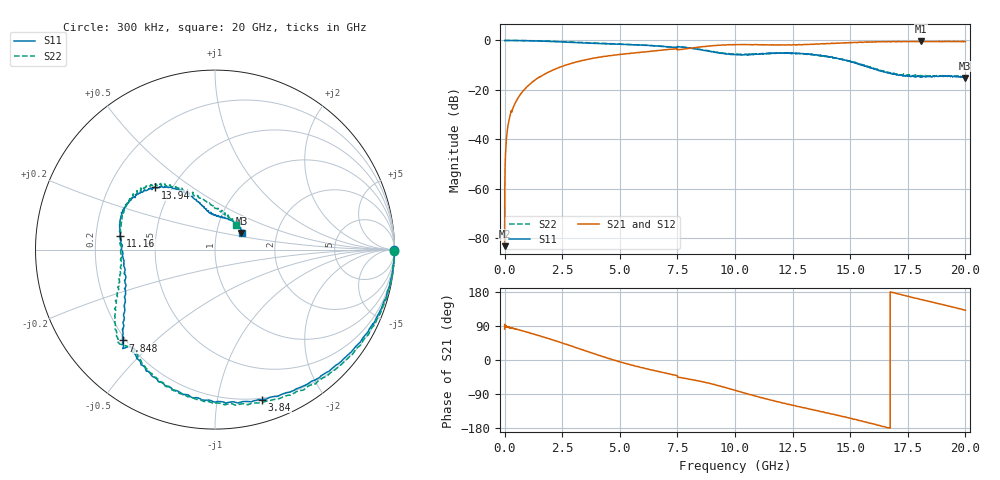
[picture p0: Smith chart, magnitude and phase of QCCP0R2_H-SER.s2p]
!{QCCP0R2}
!Johanson Technology Inc.
!www.johansontechnology.com
!Test Board Conditions:
!Substrate Type  RO4350B
!Substrate Thickness  20 mil
!Substrate Dk  3.66
!TL Type: GCPW
!TL Trace Width  36 mil
!TL Gap  12 mil
!Electrode orientation  Horizontal
!DUT TOPOLOGY	SERIES
!Mounting Pad LxW  26x36 mil
! Created Sat Jan  9 18:23:01 2021
# hz S ma R 50
! 2 Port Network Data from SP1.SP block
! freq  magS11  angS11  magS21  angS21  magS12  angS12  magS22  angS22
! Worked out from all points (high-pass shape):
!   20001 points, 300 kHz to 20 GHz, reference 50 ohm
!   highest |S21| = -0.38 dB at 18.08 GHz (marker M1); lowest = -83.3 dB at 300 kHz (marker M2)
!   |S21| within 3 dB of the highest: 7.476661 GHz to 7.499038 GHz (22.38 MHz wide, 0.299 % of centre); 7.867 GHz to end of sweep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
!   lowest |S11| = -15.2 dB at 20 GHz (marker M3), VSWR 1.42, Z = 65.9 + j12.5 ohm
!   |S11| at or under -10 dB: 15.54 GHz to end of sweep
!   |S22| runs from -14.9 to 0.0 dB; largest |S21 - S12| = 0.011
!   S11 on the Smith chart (normalised r, x): 300 kHz: open; 3.84 GHz: 0.19, -1.35; 7.848 GHz: 0.19, -0.40; 11.16 GHz: 0.30, +0.06; 13.94 GHz: 0.41, +0.36; 20 GHz: 1.32, +0.25
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300000  0.9946 -0.3  6.827e-05 81.7  9.806e-05 134.2  0.9961 -0.3
1.033e8  0.997 -1.7  0.01317 88.1  0.01316 87.8  0.9976 -1.8
1.453e8  0.9998 -2.5  0.01862 87.0  0.01853 87.3  0.9991 -2.5
2.763e8  0.9982 -4.7  0.03533 84.7  0.03533 84.6  0.9983 -4.8
5.343e8  0.9965 -8.5  0.06283 80.9  0.06278 80.9  0.9978 -8.6
9.283e8  0.9903 -15.2  0.1099 74.2  0.1099 74.3  0.9936 -15.3
1.4723e9  0.9754 -24.8  0.1779 64.6  0.1775 64.4  0.9828 -25.1
3.3343e9  0.8968 -61.9  0.3898 27.9  0.389 27.8  0.9132 -62.2
3.8403e9  0.8761 -72.5  0.4359 17.4  0.4347 17.6  0.8899 -72.7
5.2683e9  0.8303 -99.4  0.537 -9.4  0.5353 -9.1  0.8323 -99.5
6.6673e9  0.7732 -119.9  0.6267 -30.1  0.6266 -30.0  0.7679 -119.2
7.8483e9  0.7205 -135.4  0.6767 -48.4  0.6762 -48.6  0.7251 -139.4
8.8633e9  0.6055 -146.2  0.7698 -61.0  0.7687 -61.1  0.6151 -152.9
1.00003e10  0.518 -166.5  0.8233 -79.9  0.8229 -79.8  0.5296 -172.1
1.11623e10  0.5349 172.1  0.8198 -99.5  0.8204 -99.4  0.5393 167.4
1.33343e10  0.5225 142.1  0.8382 -130.6  0.8387 -130.7  0.5144 136.9
1.39443e10  0.4803 133.9  0.8598 -139.5  0.8633 -139.2  0.477 129.4
1.54183e10  0.3251 114.7  0.9246 -160.0  0.9199 -159.7  0.3382 111.5
1.66673e10  0.2188 100.1  0.9496 -179.0  0.9433 -179.0  0.2264 85.7
1.80843e10  0.1844 75.8  0.9569 159.5  0.9514 159.8  0.1944 56.8
1.99953e10  0.1738 32.1  0.9497 131.3  0.9512 131.3  0.1819 48.9
2e10  0.1743 31.9  0.9507 131.2  0.9505 131.3  0.1813 49.1
